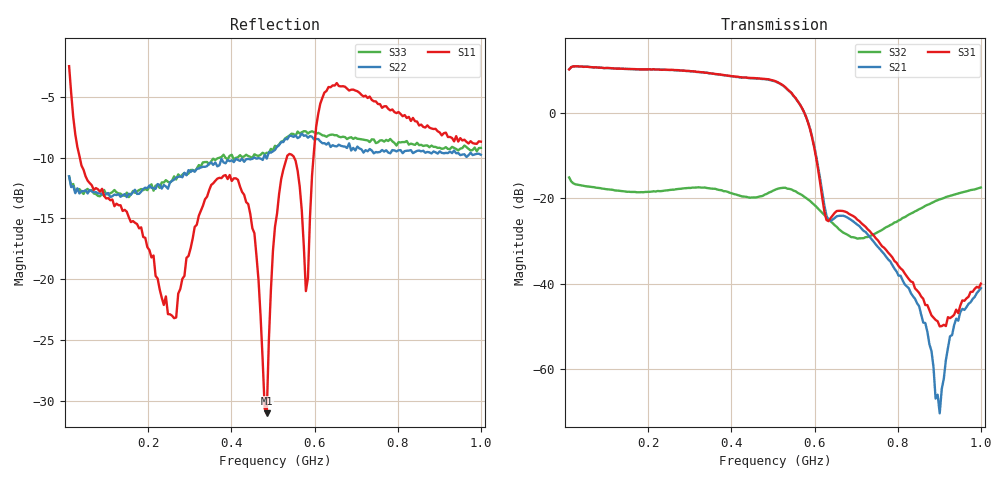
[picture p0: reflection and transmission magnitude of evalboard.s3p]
!Created with skrf (http://scikit-rf.org).
# Hz S RI R 50.0
!freq ReS11 ImS11 ReS12 ImS12 ReS13 ImS13
! ReS21 ImS21 ReS22 ImS22 ReS23 ImS23
! ReS31 ImS31 ReS32 ImS32 ReS33 ImS33
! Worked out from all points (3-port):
!   201 points, 10 MHz to 1 GHz, reference 50 ohm
!   strongest paths, dB at 10 MHz, 257.5 MHz, 505 MHz, 752.5 MHz, 1 GHz:
!     S31: 10.2, 10.1, 7.5, -29.9, -40.0
!     S21: 10.3, 10.1, 7.4, -31.4, -41.1
!     S32: -15.1, -18.0, -18.0, -27.9, -17.5
!   lowest |S11| = -31.0 dB at 485.2 MHz (marker M1), VSWR 1.06, Z = 47.5 - j1.17 ohm
!   |S11| at or under -10 dB: 35.65 MHz to 533.3 MHz (497.7 MHz wide, 175 % of centre); 550.9 MHz to 597.5 MHz (46.55 MHz wide, 8.11 % of centre)
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1e7  0.4939 -0.5648  -0.0131 -0.015  0.0131 0.0158
     3.012 1.233  -0.2526 0.0793  0.1694 -0.0523
     -2.994 -1.23  0.1692 -0.0466  -0.2453 0.0995
1.189e8  -0.1778 -0.0908  -0.00847 0.023  0.00981 -0.0222
         0.5691 -3.279  -0.1664 0.1481  0.1151 -0.0474
         -0.7128 3.25  0.1142 -0.0484  -0.1718 0.157
2.575e8  0.0689 0.0169  0.0227 0.00711  -0.0221 -0.00888
         -3.193 -0.1174  -0.0732 0.2431  0.1056 -0.0668
         3.183 0.3298  0.1064 -0.0674  -0.0926 0.2369
3.664e8  -0.2396 -0.0986  0.00867 -0.02  -0.0118 0.0191
         -0.1639 2.83  0.0653 0.2835  0.0699 -0.1039
         0.5012 -2.807  0.0685 -0.1061  0.0307 0.3123
4.852e8  -0.0253 -0.0123  -0.0195 -7.44e-05  0.0201 0.00401
         2.223 -1.087  0.1842 0.2531  0.0499 -0.1042
         -2.395 0.6903  0.0509 -0.1003  0.1798 0.2778
5.05e8  -0.1472 -0.0734  -0.0167 0.0086  0.0183 -0.0059
        1.448 -1.855  0.2005 0.2746  0.0453 -0.1174
        -1.737 1.608  0.0493 -0.1157  0.1893 0.2986
5.644e8  -0.00304 0.2407  0.00587 0.00864  -0.00373 -0.00912
         -1.147 -0.5427  0.3144 0.2217  -0.0123 -0.1111
         1.046 0.7161  -0.0194 -0.1108  0.2901 0.2711
6.8815e8  -0.0677 0.5968  4.34e-05 5.72e-05  -0.00011 -0.000419
          -0.0548 0.0101  0.3337 0.0536  -0.000722 -0.0345
          0.0625 0.0122  -0.00162 -0.035  0.3695 0.1019
9.01e8  0.3736 -0.1459  -1.91e-05 -0.000753  -0.000172 -4.98e-05
        -0.000296 5.55e-05  0.3235 -0.0881  0.0596 -0.0758
        0.00314 -0.000256  0.0592 -0.077  0.3411 -0.0632
1e9  0.0411 -0.3652  0.000369 0.000169  -0.000149 -0.000189
     -0.00868 -0.00168  0.3067 -0.1069  0.0441 -0.1292
     0.00799 0.00597  0.0464 -0.1254  0.3334 -0.0945
